TYPE RecipeEachStep :
STRUCT
	StepNo: INT;
    Completion:STRING;		//'Stable', 'Time' or 'End'
    StepTime:INT;
	AddTime:INT;
    CycleStart:BOOL;
    CycleEnd:BOOL;
    CycleNumber:INT;
	Lifter_Up:BOOL;
	AdjustTargetStepNo:INT;
	Lifter_Down:BOOL;
    LstUnit:LST;
END_STRUCT
END_TYPE
